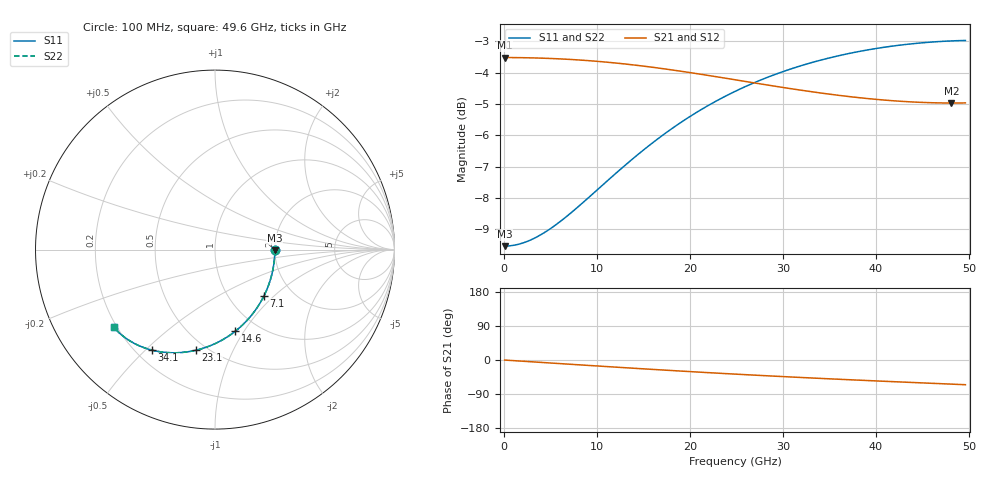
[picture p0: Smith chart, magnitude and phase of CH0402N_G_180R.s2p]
# GHz S RI R 180
! S-Parameters data
! Freq  reS11  imS11  reS21  imS21  reS12  imS12  reS22  imS22
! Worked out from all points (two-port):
!   100 points, 100 MHz to 49.6 GHz, reference 180 ohm
!   highest |S21| = -3.52 dB at 100 MHz (marker M1); lowest = -5.0 dB at 48.1 GHz (marker M2)
!   |S21| within 3 dB of the highest: start of sweep to end of sweep
!   lowest |S11| = -9.5 dB at 100 MHz (marker M3), VSWR 2.00, Z = 360 - j3.09 ohm
!   |S11| at or under -10 dB: nowhere
!   |S22| runs from -9.5 to -3.0 dB; largest |S21 - S12| = 0
!   S11 on the Smith chart (normalised r, x): 100 MHz: 2.00, -0.02; 7.1 GHz: 1.44, -0.87; 14.6 GHz: 0.78, -0.91; 23.1 GHz: 0.44, -0.73; 34.1 GHz: 0.26, -0.52; 49.6 GHz: 0.19, -0.33
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0.1  0.3333 -0.00382  0.6667 -0.00183  0.6667 -0.00183  0.3333 -0.00382
1.6  0.3301 -0.061  0.6658 -0.0293  0.6658 -0.0293  0.3301 -0.061
3.6  0.3172 -0.1357  0.6623 -0.0658  0.6623 -0.0658  0.3172 -0.1357
5.1  0.3014 -0.1897  0.6578 -0.0928  0.6578 -0.0928  0.3014 -0.1897
7.1  0.2729 -0.2577  0.6496 -0.1282  0.6496 -0.1282  0.2729 -0.2577
8.6  0.2466 -0.305  0.6417 -0.1541  0.6417 -0.1541  0.2466 -0.305
11.6  0.184 -0.3884  0.6218 -0.2038  0.6218 -0.2038  0.184 -0.3884
14.6  0.1118 -0.4556  0.597 -0.2498  0.597 -0.2498  0.1118 -0.4556
16.6  0.0608 -0.4913  0.5781 -0.278  0.5781 -0.278  0.0608 -0.4913
19.6  -0.0173 -0.5317  0.5474 -0.3163  0.5474 -0.3163  -0.0173 -0.5317
21.1  -0.0561 -0.5464  0.5312 -0.3336  0.5312 -0.3336  -0.0561 -0.5464
23.1  -0.107 -0.5609  0.509 -0.3548  0.509 -0.3548  -0.107 -0.5609
25.1  -0.1564 -0.57  0.4865 -0.374  0.4865 -0.374  -0.1564 -0.57
27.1  -0.2037 -0.5744  0.4639 -0.3912  0.4639 -0.3912  -0.2037 -0.5744
29.1  -0.2487 -0.5746  0.4414 -0.4067  0.4414 -0.4067  -0.2487 -0.5746
33.1  -0.3312 -0.5645  0.3974 -0.4333  0.3974 -0.4333  -0.3312 -0.5645
34.1  -0.3502 -0.5602  0.3867 -0.4392  0.3867 -0.4392  -0.3502 -0.5602
37.6  -0.4114 -0.5403  0.3503 -0.4579  0.3503 -0.4579  -0.4114 -0.5403
41.6  -0.4717 -0.5102  0.3108 -0.4768  0.3108 -0.4768  -0.4717 -0.5102
44.6  -0.5102 -0.4836  0.2824 -0.4901  0.2824 -0.4901  -0.5102 -0.4836
48.1  -0.5484 -0.449  0.2502 -0.5056  0.2502 -0.5056  -0.5484 -0.449
49.6  -0.5625 -0.4331  0.2366 -0.5123  0.2366 -0.5123  -0.5625 -0.4331
